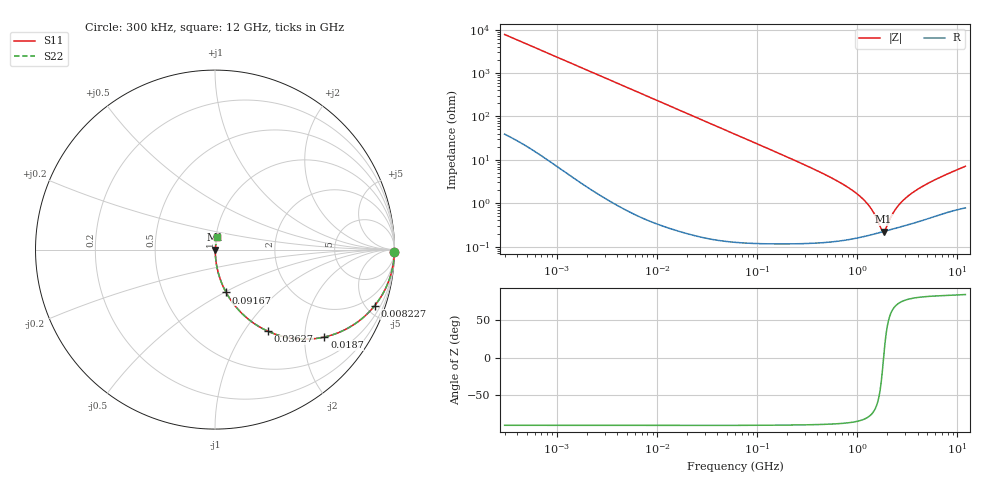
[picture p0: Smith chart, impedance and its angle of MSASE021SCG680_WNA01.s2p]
! MSASE021SCG680_WNA01  S-PARAMETER MODEL  ( Standard Model )
! Model Generated by TAIYO YUDEN Corporation (http://www.ty-top.com)
! Version 1.0
! TAIYO YUDEN Control No. 241126
! Copyright(c) 2024 TAIYO YUDEN CO.,LTD. All Rights Reserved.
! Product Description (link to TY-COMPAS)
! https://ds.yuden.co.jp/TYCOMPAS/or/detail?pn=MSASE021SCG680GWNA01&u=M
! Products Name : Multilayer Ceramic Capacitors
! Characteristics :
!  Capacitance : 68 [pF] , Rated Voltage : 16 [V] , TCC : CG / C0G
!  Case Size : 0.25 x 0.125 / 0.0098 x 0.0049 [mm/inch] , Thickness : 0.125 / 0.0049 [mm/inch]
!  (Conditions: Temperature = 25 [degC] , DC Bias Voltage = 0 [V])
! External Node Assignments :
!  1  o---| |---o  2
! GND o---------o GND
! Frequency Range : 0.3MHz  -  12000MHz  [ 401 STEP ]
# MHZ S RI R 50
! Freq[MHz].  S11 Real  S11 Imag  S21 Real  S21 Imag  S12 Real  S12 Imag  S22 Real  S22 Imag
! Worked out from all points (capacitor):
!   401 points, 300 kHz to 12 GHz, reference 50 ohm
!   read as one part in series: C = 68.4 pF near 316.3 kHz
!   lowest |Z| = 222 mohm at 1.829 GHz (marker M1)
!   series resonance near 1.829 GHz, so ESL is about 110 pH
!   S11 on the Smith chart (normalised r, x): 300 kHz: open; 8.227 MHz: 1.01, -5.68; 18.7 MHz: 1.00, -2.50; 36.27 MHz: 1.00, -1.29; 91.67 MHz: 1.00, -0.51; 12 GHz: 1.02, +0.14
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0.3  0.9998 -0.0129  0.000231 0.0129  0.000231 0.0129  0.9998 -0.0129
1.769972  0.9941 -0.0753  0.00587 0.0753  0.00587 0.0753  0.9941 -0.0753
3.918509  0.9724 -0.163  0.0276 0.163  0.0276 0.163  0.9724 -0.163
8.227445  0.8895 -0.3128  0.1105 0.3128  0.1105 0.3128  0.8895 -0.3128
10.44266  0.8334 -0.3719  0.1666 0.3719  0.1666 0.3719  0.8334 -0.3719
18.70358  0.6098 -0.487  0.3902 0.487  0.3902 0.487  0.6098 -0.487
36.27049  0.2941 -0.4545  0.7059 0.4545  0.7059 0.4545  0.2941 -0.4545
60  0.1326 -0.3375  0.8674 0.3375  0.8674 0.3375  0.1326 -0.3375
91.67136  0.0619 -0.2386  0.9381 0.2386  0.9381 0.2386  0.0619 -0.2386
353.9943  0.00519 -0.0631  0.9948 0.0631  0.9948 0.0631  0.00519 -0.0631
686.4755  0.00219 -0.0289  0.9978 0.0289  0.9978 0.0289  0.00219 -0.0289
1048.836  0.00183 -0.0147  0.9982 0.0147  0.9982 0.0147  0.00183 -0.0147
1366.97  0.00191 -0.00734  0.9981 0.00734  0.9981 0.00734  0.00191 -0.00734
1735.023  0.00215 -0.0013  0.9979 0.0013  0.9979 0.0013  0.00215 -0.0013
1829.429  0.00222 1.01e-06  0.9978 -1.01e-06  0.9978 -1.01e-06  0.00222 1.01e-06
1928.972  0.00229 0.0013  0.9977 -0.0013  0.9977 -0.0013  0.00229 0.0013
2088.533  0.00242 0.00324  0.9976 -0.00324  0.9976 -0.00324  0.00242 0.00324
2321.999  0.00261 0.00584  0.9974 -0.00584  0.9974 -0.00584  0.00261 0.00584
2581.562  0.00282 0.00848  0.9972 -0.00848  0.9972 -0.00848  0.00282 0.00848
3547.679  0.00367 0.0169  0.9963 -0.0169  0.9963 -0.0169  0.00367 0.0169
5868.704  0.00599 0.0334  0.994 -0.0334  0.994 -0.0334  0.00599 0.0334
12000  0.0126 0.0693  0.9874 -0.0693  0.9874 -0.0693  0.0126 0.0693
